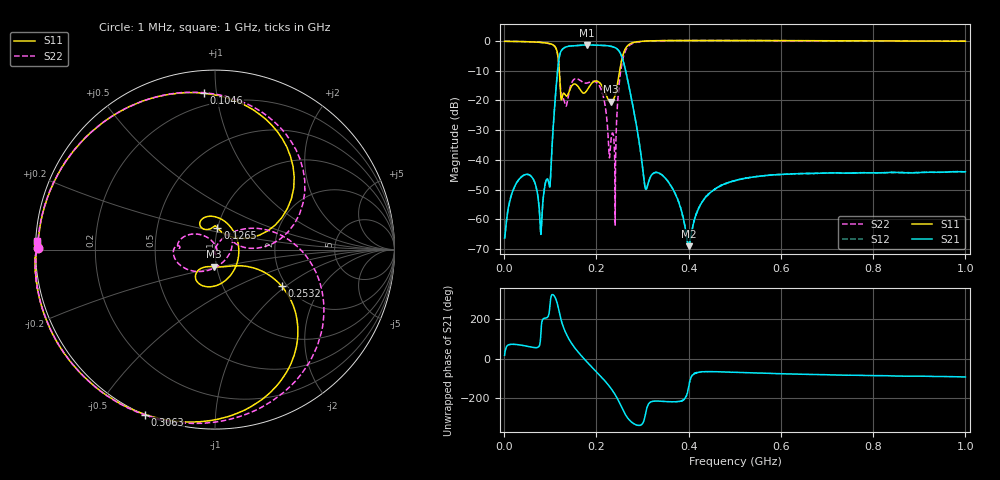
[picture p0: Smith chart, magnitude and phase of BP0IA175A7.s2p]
!Agilent Technologies,E8358A,US41080443,A.07.50.56
!Agilent E8358A: A.07.50.56
!Date: Tuesday, October 31, 2017 22:07:42
!Correction: S11(Full 2 Port(1,2))
!S21(Full 2 Port(1,2))
!S12(Full 2 Port(1,2))
!S22(Full 2 Port(1,2))
!S2P File: Measurements: S11, S21, S12, S22:
# Hz S  dB  R 50
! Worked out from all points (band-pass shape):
!   1601 points, 1 MHz to 1 GHz, reference 50 ohm
!   highest |S21| = -1.32 dB at 180.2 MHz (marker M1); lowest = -69.0 dB at 400.6 MHz (marker M2)
!   |S21| within 3 dB of the highest: 121.2 MHz to 252.6 MHz (131.4 MHz wide, 70.3 % of centre)
!   lowest |S11| = -20.4 dB at 230.8 MHz (marker M3), VSWR 1.21, Z = 48.6 - j9.36 ohm
!   |S11| at or under -10 dB: 119.6 MHz to 250.3 MHz (130.7 MHz wide, 70.7 % of centre)
!   |S22| runs from -61.9 to 0.2 dB; largest |S21 - S12| = 0.0046
!   S11 on the Smith chart (normalised r, x): 1 MHz: 0.01, +0.00; 104.6 MHz: 0.13, +0.92; 126.5 MHz: 1.00, +0.24; 253.2 MHz: 1.88, -0.93; 306.3 MHz: 0.00, -0.66; 1 GHz: 0.00, +0.02
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1000000  -0.12 179.6  -66.26 16.7  -66.53 16.6  -0.10 179.5
4.34575e7  -0.22 159.5  -45.08 64.9  -45.08 64.8  -0.21 159.4
8.029562e7  -0.48 133.1  -63.67 153.8  -64.03 155.2  -0.49 132.4
1.046462e8  -1.18 94.1  -33.29 -37.7  -33.29 -37.4  -1.24 90.1
1.190069e8  -8.84 22.1  -5.94 -120.8  -5.93 -120.6  -8.68 9.2
1.264994e8  -18.36 83.4  -2.75 171.1  -2.74 171.4  -19.23 32.8
1.427331e8  -16.29 122.0  -1.71 89.1  -1.68 89.3  -15.80 -131.5
1.677081e8  -16.99 38.3  -1.41 12.9  -1.39 12.8  -13.60 174.0
1.801956e8  -16.45 -41.1  -1.32 -18.9  -1.33 -19.0  -14.12 177.7
2.101656e8  -14.61 -125.9  -1.45 -91.1  -1.49 -91.1  -16.25 145.9
2.3077e8  -20.40 -93.1  -1.74 -148.2  -1.76 -148.1  -34.66 -47.8
2.413844e8  -17.80 -45.1  -2.30 175.0  -2.32 175.0  -42.00 69.4
2.532475e8  -7.48 -28.7  -4.56 121.7  -4.61 121.8  -9.46 17.2
2.769738e8  -0.67 -83.7  -20.20 38.2  -20.23 38.6  -0.93 -68.7
3.063194e8  -0.02 -112.9  -49.72 80.0  -49.65 79.6  -0.07 -106.6
3.344162e8  0.10 -127.0  -44.39 145.2  -44.39 145.5  0.09 -123.6
4.006e8  0.17 -144.7  -69.03 -140.2  -68.51 -142.5  0.16 -143.7
4.336919e8  0.17 -150.1  -53.20 -66.7  -53.17 -67.0  0.17 -149.6
5.005e8  0.16 -157.8  -46.99 -69.1  -47.01 -69.3  0.14 -158.0
6.672081e8  0.10 -169.6  -44.56 -80.3  -44.60 -80.2  0.08 -170.1
8.339162e8  0.02 -176.9  -44.24 -87.1  -44.21 -87.1  0.01 -177.5
1e9  -0.08 177.6  -44.01 -93.0  -44.06 -92.8  -0.08 177.2
